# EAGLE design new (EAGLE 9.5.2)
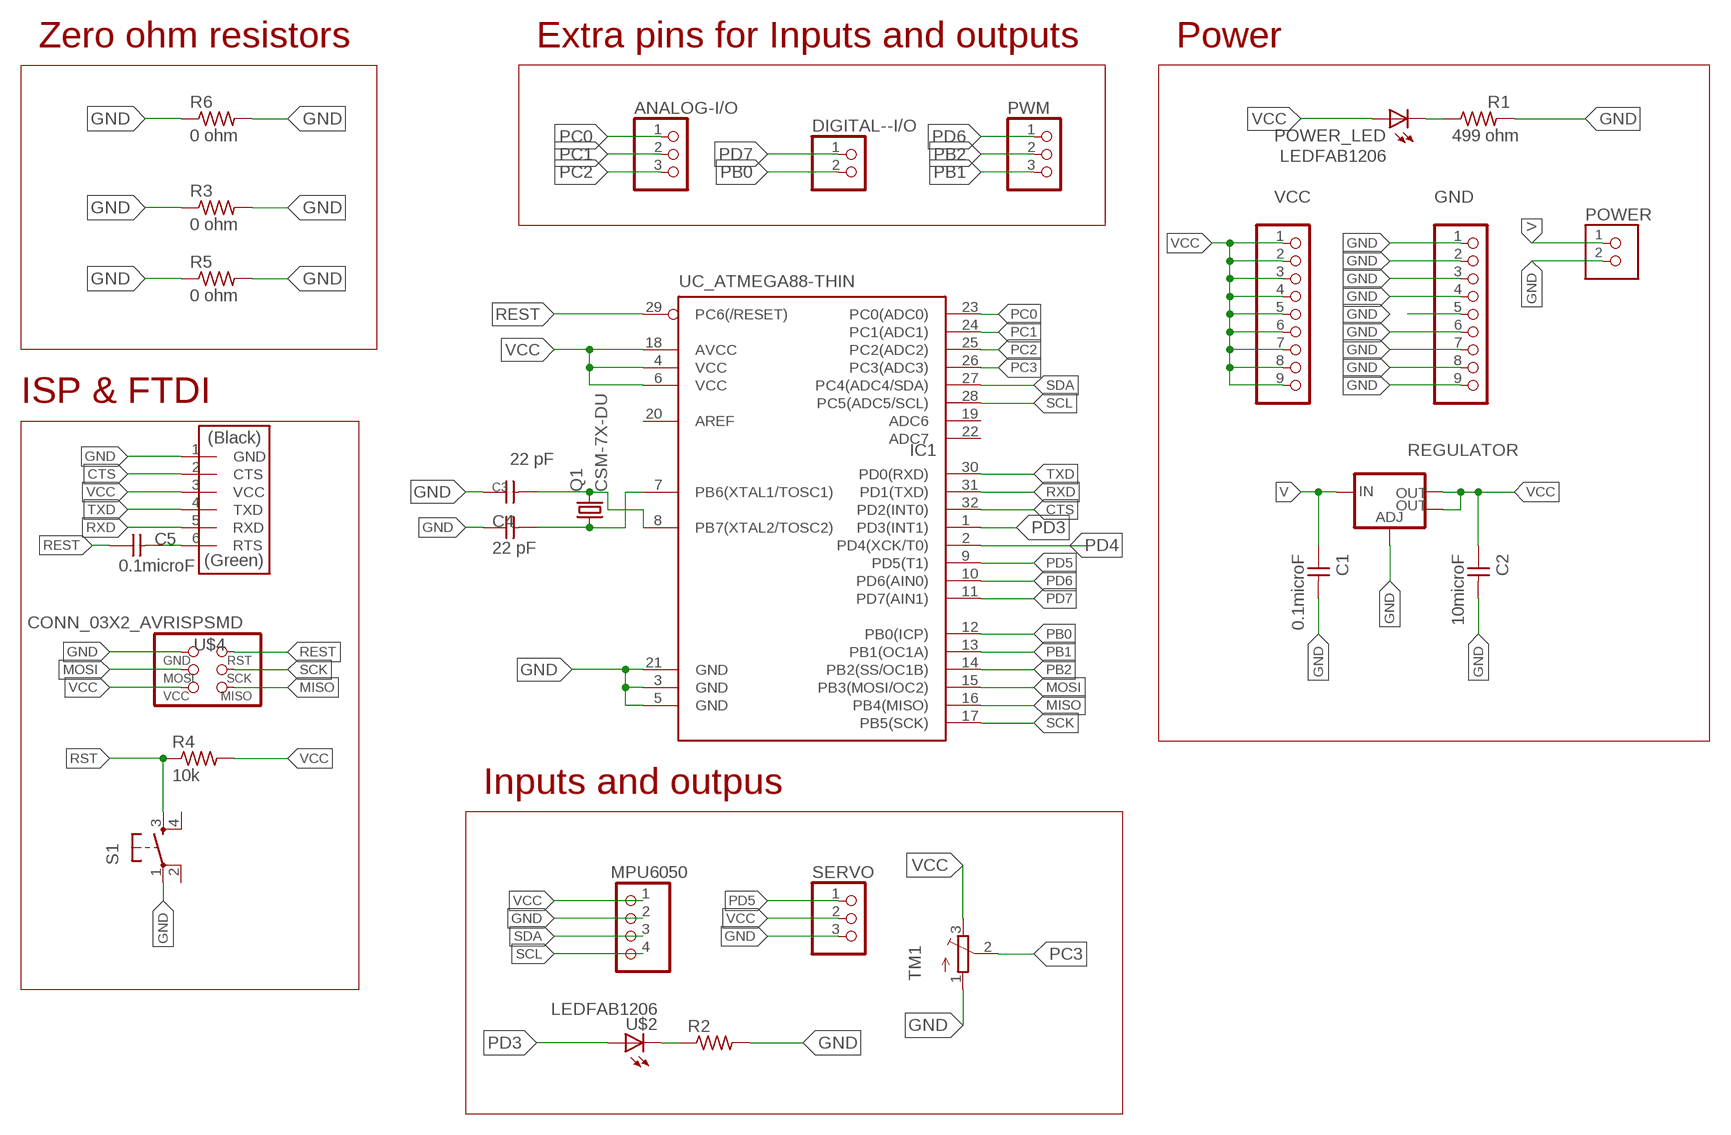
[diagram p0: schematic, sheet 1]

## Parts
ANALOG-I/O  PINHD-1X3  [1X03]
C1  0.1microF  CAP_UNPOLARIZEDFAB  [C1206FAB]
C2  10microF  CAP_UNPOLARIZEDFAB  [C1206FAB]
C3  22 pF  CAP_UNPOLARIZEDFAB  [C1206FAB]
C4  22 pF  CAP_UNPOLARIZEDFAB  [C1206FAB]
C5  0.1microF  CAP_UNPOLARIZEDFAB  [C1206FAB]
DIGITAL--I/O  PINHD-1X2  [1X02]
GND  PINHD-1X9  [1X09]
IC1  UC_ATMEGA88-THIN  [TQFP32-08THIN]
MPU6050  PINHD-1X4  [1X04]
POWER  CONN_02_TERM-FABLAB  [ED555DS-2DS]
POWER_LED  LEDFAB1206  [LED1206FAB]
PWM  PINHD-1X3  [1X03]
Q1  CSM-7X-DU  [CSM-7X-DU]
R1  499 ohm  R1206FAB  [R1206FAB]
R2  R1206FAB  [R1206FAB]
R3  0 ohm  R1206FAB  [R1206FAB]
R4  10k  R1206FAB  [R1206FAB]
R5  0 ohm  R1206FAB  [R1206FAB]
R6  0 ohm  R1206FAB  [R1206FAB]
REGULATOR  VR_REGULATOR_LM1117SOT223  [SOT223]
S1  SW_SWITCH_TACTILE_6MM6MM_SWITCH  [6MM_SWITCH]
SERVO  PINHD-1X3  [1X03]
TM1  TRIMPOTTC33X  [TC33X]
U$1  CONN_06_FTDI-SMD-HEADER  [1X06SMD]
U$2  LEDFAB1206  [LED1206FAB]
U$4  CONN_03X2_AVRISPSMD  [2X03SMD]
VCC  PINHD-1X9  [1X09]

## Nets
CTS: IC1.32(PD2(INT0)) U$1.2(CTS)
GND: C1.2 C2.2 C3.1 C4.1 GND.1 GND.2 GND.3 GND.4 GND.5 GND.6 GND.7 GND.8 GND.9 IC1.3(GND) IC1.5(GND) IC1.21(GND) MPU6050.2 POWER.2 R1.2 R2.2 R3.1 R3.2 R5.1 R5.2 R6.1 R6.2 REGULATOR.1(ADJ) S1.1(P) SERVO.3 TM1.1(A) U$1.1(GND) U$4.6(GND)
MISO: IC1.16(PB4(MISO)) U$4.1(MISO)
MOSI: IC1.15(PB3(MOSI/OC2)) U$4.4(MOSI)
N$1: C5.2 U$1.6(RTS)
N$2: R2.1 U$2.2(C)
N$3: POWER_LED.2(C) R1.1
N$4: C3.2 IC1.8(PB7(XTAL2/TOSC2)) Q1.2
N$5: C4.2 IC1.7(PB6(XTAL1/TOSC1)) Q1.1
PB0: DIGITAL--I/O.2 IC1.12(PB0(ICP))
PB1: IC1.13(PB1(OC1A)) PWM.3
PB2: IC1.14(PB2(SS/OC1B)) PWM.2
PC0: ANALOG-I/O.1 IC1.23(PC0(ADC0))
PC1: ANALOG-I/O.2 IC1.24(PC1(ADC1))
PC2: ANALOG-I/O.3 IC1.25(PC2(ADC2))
PC3: IC1.26(PC3(ADC3)) TM1.2(S)
PD3: IC1.1(PD3(INT1)) U$2.1(A)
PD4: IC1.2(PD4(XCK/T0))
PD5: IC1.9(PD5(T1)) SERVO.1
PD6: IC1.10(PD6(AIN0)) PWM.1
PD7: DIGITAL--I/O.1 IC1.11(PD7(AIN1))
REST: C5.1 IC1.29(PC6(/RESET)) U$4.5(RST)
RST: R4.1 S1.3(S)
RXD: IC1.31(PD1(TXD)) U$1.5(RXD)
SCK: IC1.17(PB5(SCK)) U$4.3(SCK)
SCL: IC1.28(PC5(ADC5/SCL)) MPU6050.4
SDA: IC1.27(PC4(ADC4/SDA)) MPU6050.3
TXD: IC1.30(PD0(RXD)) U$1.4(TXD)
V: C1.1 POWER.1 REGULATOR.3(IN)
VCC: C2.1 IC1.4(VCC) IC1.6(VCC) IC1.18(AVCC) MPU6050.1 POWER_LED.1(A) R4.2 REGULATOR.2(OUT) REGULATOR.4(OUT) SERVO.2 TM1.3(E) U$1.3(VCC) U$4.2(VCC) VCC.1 VCC.2 VCC.3 VCC.4 VCC.5 VCC.6 VCC.7 VCC.8 VCC.9
Unconnected: IC1.19(ADC6) IC1.20(AREF) IC1.22(ADC7) S1.2(P1) S1.4(S1)

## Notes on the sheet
- Zero ohm resistors | Extra pins for Inputs and outputs | Power
- ISP & FTDI
- Inputs and outpus

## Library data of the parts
ANALOG-I/O PWM SERVO = pinhead:PINHD-1X3: PIN HEADER
C1-C5 = eagle_fab:CAP_UNPOLARIZED
DIGITAL--I/O = pinhead:PINHD-1X2: PIN HEADER
GND VCC = pinhead:PINHD-1X9: PIN HEADER
IC1 = eagle_fab:UC_ATMEGA88-THIN
MPU6050 = pinhead:PINHD-1X4: PIN HEADER
POWER = eagle_fab:CONN_02_TERM: 3.5mm terminal block, 2 positions ED555-2DS as found in the fablab inventory.
POWER_LED U$2 = eagle_fab:LED: LED
Q1 = crystal-2:CSM-7X-DU: SMD CRYSTAL; OC_FARNELL: unknown; OC_NEWARK: unknown
R1-R6 = eagle_fab:R: Resistor (US Symbol)
REGULATOR = eagle_fab:VR_REGULATOR_LM1117: Voltage Regulator LM1117 Standard adjustable voltage regulator but in SMD form. Spark Fun Electronics SKU : COM-00595; PROD_ID: VREG-08170
S1 = eagle_fab:SW_SWITCH_TACTILE_6MM: OMRON SWITCH
TM1 = ada1:TRIMPOT: SMT trimmer potentiometer part number TC33X http://www.ladyada.net/library/eagle
U$1 = eagle_fab:CONN_06_FTDI-SMD-HEADER
U$4 = eagle_fab:CONN_03X2_AVRISP

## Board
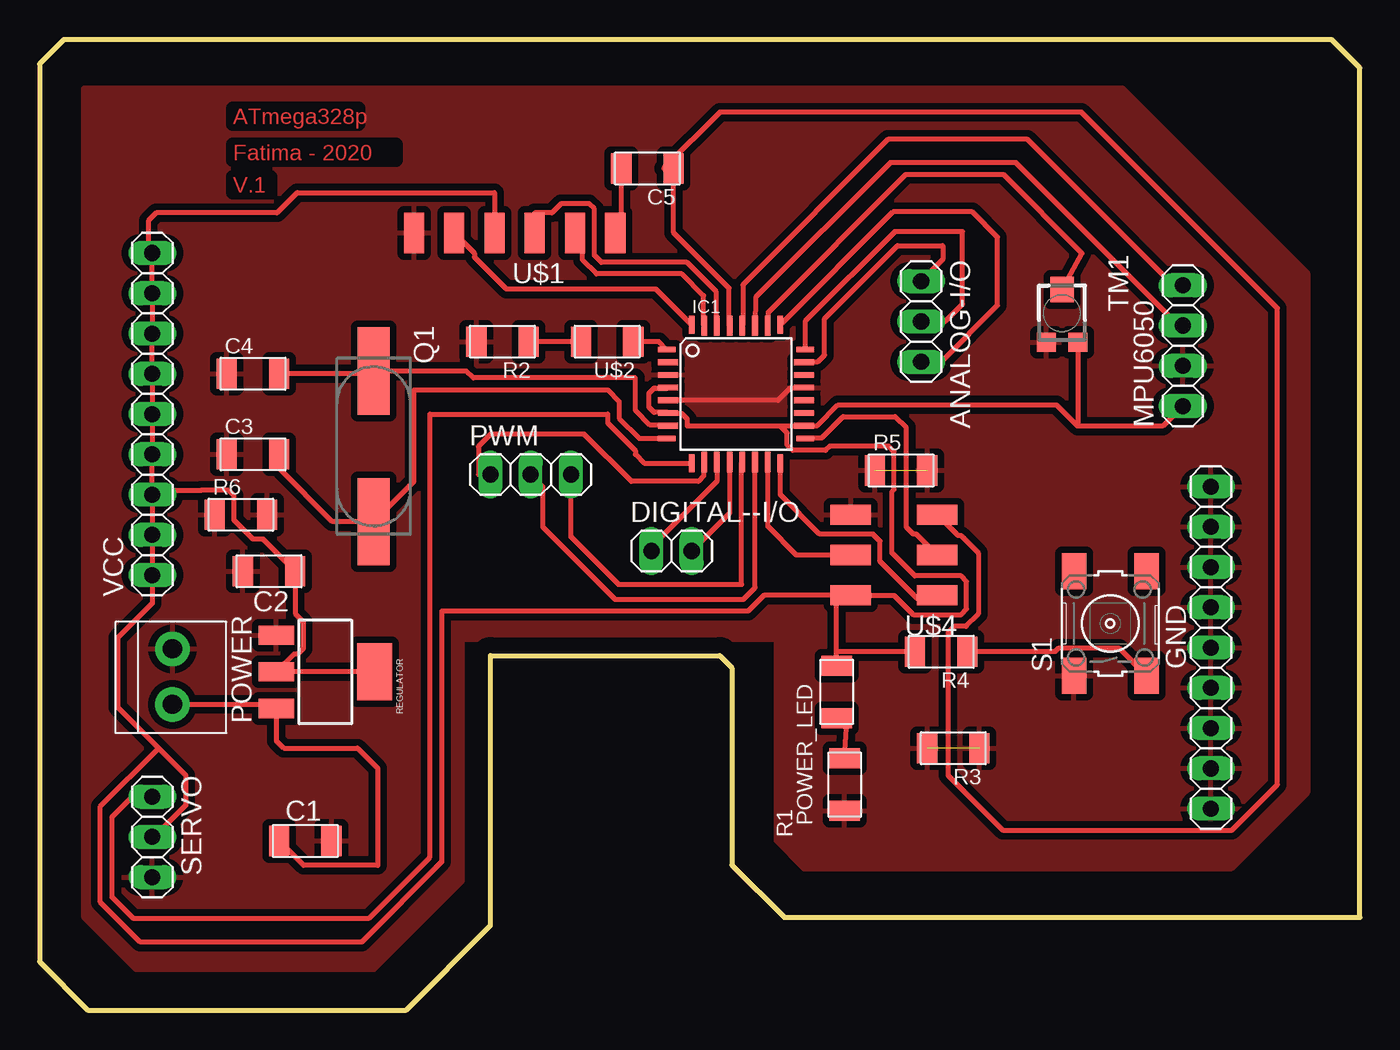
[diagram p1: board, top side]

Size 83.31 x 61.21 mm. Coordinates in mm from the lower left corner, seen from the top.
Outline: 81.53,61.21 1.52,61.21 0,59.69 0,3.05 3.05,0 23.11,0 28.45,5.33 28.45,22.35 42.93,22.35 43.69,21.59 43.69,9.14 46.99,5.84 83.31,5.84 83.31,59.44 81.53,61.21
Copper layers (1*16): Top 0.035mm / dielectric 1.5mm / Bottom 0.035mm
Design rules "default *": minimum track width 12mil, minimum drill 0.35mm, track to track 17mil, track to pad 17mil, pad to pad 17mil, via to via 17mil, smd to smd 17mil, copper to edge 40mil, drill to drill 6mil, minimum pad ring 10mil, minimum via ring 8mil, stop-mask expansion 4mil, vias tented up to drill 0mil, thermal gap 17mil

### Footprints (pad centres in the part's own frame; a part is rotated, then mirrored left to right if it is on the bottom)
1X03 = drill 1.016 long: 1 -2.54,0; 2 0,0; 3 2.54,0
C1206FAB = smd 1.27 x 1.905: 1 -1.651,0; 2 1.651,0
1X02 = drill 1.016 long: 1 -1.27,0; 2 1.27,0
1X09 = drill 1.016 long: 1 -10.16,0; 2 -7.62,0; 3 -5.08,0; 4 -2.54,0; 5 0,0; 6 2.54,0; 7 5.08,0; 8 7.62,0; 9 10.16,0
TQFP32-08THIN = smd 1.118 x 0.356: 1 -4.369,2.8; 8 -4.369,-2.8; 17 4.369,-2.8; 24 4.369,2.8 | smd 1.27 x 0.356: 2 -4.293,2; 3 -4.293,1.2; 4 -4.293,0.4; 5 -4.293,-0.4; 6 -4.293,-1.2; 7 -4.293,-2; 18 4.293,-2; 19 4.293,-1.2; 20 4.293,-0.4; 21 4.293,0.4; 22 4.293,1.2; 23 4.293,2 | smd 0.356 x 1.118: 9 -2.8,-4.369; 16 2.8,-4.369; 25 2.8,4.369; 32 -2.8,4.369 | smd 0.356 x 1.27: 10 -2,-4.293; 14 1.2,-4.293; 15 2,-4.293; 26 2,4.293; 27 1.2,4.293; 31 -2,4.293 | smd 0.35 x 1.27: 11 -1.2,-4.293; 12 -0.4,-4.293; 13 0.4,-4.293; 28 0.4,4.293; 29 -0.4,4.293; 30 -1.2,4.293
1X04 = drill 1.016 long: 1 -3.81,0; 2 -1.27,0; 3 1.27,0; 4 3.81,0
ED555DS-2DS = drill 1.2 pad 2.184: 1 1.8,0; 2 -1.7,0
LED1206FAB = smd 1.27 x 1.905: 1 -1.651,0; 2 1.651,0
CSM-7X-DU = smd 5.5 x 2: 1 -4.75,0; 2 4.75,0
R1206FAB = smd 1.27 x 1.905: 1 -1.651,0; 2 1.651,0
SOT223 = smd 1.219 x 2.235: 1 -2.311,-3.099; 2 0,-3.099; 3 2.311,-3.099 | smd 3.6 x 2.2: 4 0,3.099
6MM_SWITCH = smd 2.286 x 1.524: 1 -3.302,2.286; 2 3.302,2.286; 3 -3.302,-2.286; 4 3.302,-2.286
TC33X = smd 1.2 x 1.2: 1 -1,-1.825; 3 1,-1.825 | smd 1.5 x 1.6: 2 0,1.5
1X06SMD = smd 2.54 x 1.27: 1 0,6.35; 2 0,3.81; 3 0,1.27; 4 0,-1.27; 5 0,-3.81; 6 0,-6.35
2X03SMD = smd 2.54 x 1.27: 1 -2.54,2.54; 2 2.92,2.54; 3 -2.54,0; 4 2.92,0; 5 -2.54,-2.54; 6 2.92,-2.54

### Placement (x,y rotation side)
ANALOG-I/O  55.63,43.43 270 top
C1  16.76,10.67 0 top
C2  14.48,27.69 180 top
C3  13.46,35.05 0 top
C4  13.46,40.13 0 top
C5  38.35,53.09 180 top
DIGITAL--I/O  39.88,28.96 0 top
GND  73.91,22.86 90 top
IC1  43.94,38.86 0 top
MPU6050  72.14,41.91 90 top
POWER  8.38,21.08 270 top
POWER_LED  50.29,20.07 270 top
PWM  30.99,33.78 0 top
Q1  21.08,35.56 270 top
R1  50.8,14.22 270 top
R2  29.21,42.16 180 top
R3  57.66,16.51 180 top
R4  56.9,22.61 180 top
R5  54.36,34.04 0 top
R6  12.7,31.24 0 top
REGULATOR  18.03,21.34 270 top
S1  67.56,24.38 90 top
SERVO  7.11,10.92 270 top
TM1  64.52,43.94 0 top
U$1  29.97,49.02 90 top
U$2  35.81,42.16 180 top
U$4  54.1,28.7 180 top
VCC  7.11,37.59 90 top

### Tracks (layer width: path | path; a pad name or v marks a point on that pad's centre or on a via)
CTS
  Top 0.305: IC1.32 38.89,45.48 29.45,45.48 27.43,47.5 27.43,47.75 U$1.2
GND  (2 unrouted)
  Top 0.305: 12.19,40.13 C4.1 | 12.19,35.05 C3.1 | IC1.21 48.2,39.22 47.36,39.22 46.6,38.46 IC1.5 | 50.7,31.72 U$4.6
  pour Top: 2.79,58.17 68.33,58.17 80.01,46.48 80.01,13.72 75.18,8.89 48.26,8.89 46.48,10.67 46.48,23.37 26.67,23.37 26.67,8.13 21.08,2.54 6.1,2.54 2.79,5.84
MISO
  Top 0.305: U$4.1 56.44,25.96 55.38,25.96 53.04,28.31 53.04,29.58 52.59,30.02 49.23,30.02 46.74,32.51 IC1.16
MOSI
  Top 0.305: IC1.15 45.94,31.43 45.95,31.43 45.95,30.5 47.75,28.7 U$4.4
N$1
  Top 0.305: C5.2 36.7,49.4 U$1.6
N$2
  Top 0.305: U$2.2 R2.1
N$3
  Top 0.305: POWER_LED.2 50.93,17.78 R1.1
N$4
  Top 0.305: IC1.8 37.85,36.06 36.58,37.34 36.58,38.38 35.84,39.12 23.62,39.12 23.62,33.35 Q1.2 18.47,30.81 15.11,34.16 C3.2
N$5
  Top 0.305: C4.2 20.9,40.13 Q1.1 26.92,40.31 27.36,39.88 37.59,39.88 37.59,37.84 38.53,36.9 39.61,36.9 IC1.7
PB0
  Top 0.305: DIGITAL--I/O.2 43.54,31.35 IC1.12
PB1
  Top 0.305: IC1.13 44.3,34.53 44.3,26.85 36.53,26.85 33.53,29.85 PWM.3
PB2
  Top 0.305: PWM.2 31.75,33.02 31.75,30.48 36.32,25.91 44.4,25.91 45.14,26.65 IC1.14
PC0
  Top 0.305: IC1.23 48.27,40.9 49.11,40.9 49.53,41.32 49.53,43.62 54.14,48.23 57,48.23 57,47.35 ANALOG-I/O.1
PC1
  Top 0.305: ANALOG-I/O.2 57.15,43.43 58.24,44.53 58.24,49.1 53.97,49.1 48.31,43.44 IC1.24
PC2
  Top 0.305: ANALOG-I/O.3 56.9,40.89 60.45,44.45 60.45,48.75 58.86,50.34 53.85,50.34 IC1.25
PC3
  Top 0.305: IC1.26 45.98,43.19 45.98,44.03 54.66,52.71 60.8,52.71 65.78,47.73 TM1.2
PD3
  Top 0.305: IC1.1 39.07,42.16 U$2.1
PD5
  Top 0.305: SERVO.1 5.84,13.46 4.57,12.19 4.57,7.11 5.89,5.79 20.78,5.79 24.64,9.65 24.64,37.59 35.84,37.59 35.84,37.03 37.59,35.28 37.59,35.05 38.15,34.49 IC1.9
PD6
  Top 0.305: IC1.10 41.9,34.53 41.9,33.69 41.56,33.35 37.34,33.35 34.37,36.32 28.45,36.32 27.69,35.56 27.69,33.78 PWM.1
PD7
  Top 0.305: DIGITAL--I/O.1 38.61,29.21 42.74,33.34 IC1.11
REST
  Top 0.305: IC1.29 43.5,43.2 43.5,45.55 40.01,49.04 40.01,52.83 | 40.01,52.83 C5.1 | 40.01,52.83 39.62,52.83 39.37,53.09 42.93,56.64 65.74,56.64 78.11,44.27 78.11,14.23 75.23,11.35 60.78,11.35 57.33,14.81 57.33,23.8 57.73,24.21 58.46,24.21 59.23,24.98 59.23,28.84 58.15,29.92 57.96,29.92 U$4.5
RST
  Top 0.305: R4.1 64.07,22.61 64.27,22.81 68.12,22.81 S1.3
RXD
  Top 0.305: IC1.31 41.9,43.19 41.9,45.06 40.53,46.43 35.14,46.43 34.27,47.31 34.27,48.54 U$1.5
SCK
  Top 0.305: 57.12,28.22 U$4.3 55.32,30.02 55.13,30.02 54.69,30.47 54.69,36.75 54,37.44 50.69,37.44 49.35,36.1 48.35,36.1 IC1.17
SCL
  Top 0.305: IC1.28 44.38,43.19 44.38,45.75 53.54,54.91 62.33,54.91 71.53,45.72 MPU6050.4
SDA
  Top 0.305: MPU6050.3 72.01,43.05 61.61,53.45 53.68,53.45 45.18,44.95 IC1.27
TXD
  Top 0.305: IC1.30 42.7,43.19 42.7,45.3 40.84,47.17 35.45,47.17 35,47.61 35,50.53 34.66,50.88 32.91,50.88 32.32,50.29 31.24,50.29 U$1.4
V
  Top 0.305: POWER.1 14.68,19.28 REGULATOR.3 14.94,16.99 15.41,16.52 20.05,16.52 21.34,15.24 21.34,9.13 16.65,9.13 C1.1
VCC
  Top 0.305: 7.11,47.5 VCC.8 VCC.7 VCC.6 VCC.5 VCC.4 7.11,32.77 | 7.11,47.5 VCC.9 | IC1.4 39.62,39.24 38.86,39.24 38.85,39.22 38.77,39.22 38.43,38.88 38.43,38.04 38.77,37.7 39.61,37.7 IC1.6 40.06,37.66 40.1,37.62 40.53,37.62 40.87,37.28 40.87,36.85 40.89,36.83 46.68,36.83 46.69,36.84 46.74,36.84 | 46.74,36.84 48.21,36.84 IC1.18 49.07,36.86 50.39,38.18 64.17,38.18 65.52,36.83 | 7.11,32.77 VCC.3 VCC.2 VCC.1 7.11,25.66 4.93,23.48 4.93,19.1 7.44,16.58 | SERVO.2 7.24,10.92 9.22,12.9 9.22,14.8 7.44,16.58 | U$1.3 28.7,51.56 16.26,51.56 14.99,50.29 7.37,50.29 6.86,49.78 6.86,47.75 7.11,47.5 | REGULATOR.4 REGULATOR.2 16.05,22.45 16.29,22.45 16.64,22.8 16.64,24.5 16.13,25.01 C2.1 14.11,29.7 13.47,29.7 12.27,30.91 12.27,32.44 11.93,32.78 10.17,32.78 10.16,32.77 7.11,32.77 | U$4.2 50.29,26.16 50.29,22.61 | POWER_LED.1 50.29,22.61 | MPU6050.1 70.87,36.83 65.52,36.83 | TM1.3 65.52,36.83 | R4.2 50.29,22.61 | U$4.2 45.7,26.16 44.71,25.17 25.38,25.17 25.38,9.35 20.32,4.29 6.35,4.29 3.83,6.81 3.83,12.85 7.44,16.45 7.44,16.58 | U$4.2 53.91,26.16 55.13,24.94 58.15,24.94 58.5,25.29 58.5,27.04 58.15,27.38 55.23,27.38 53.77,28.84 53.77,32.69 53.92,32.84 53.92,35.23 53.58,35.57 49.87,35.57 49.59,35.3 47.51,35.3 47.17,35.64 47.17,36.41 46.74,36.84

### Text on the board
Top: ATmega328p | Fatima - 2020 | V.1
